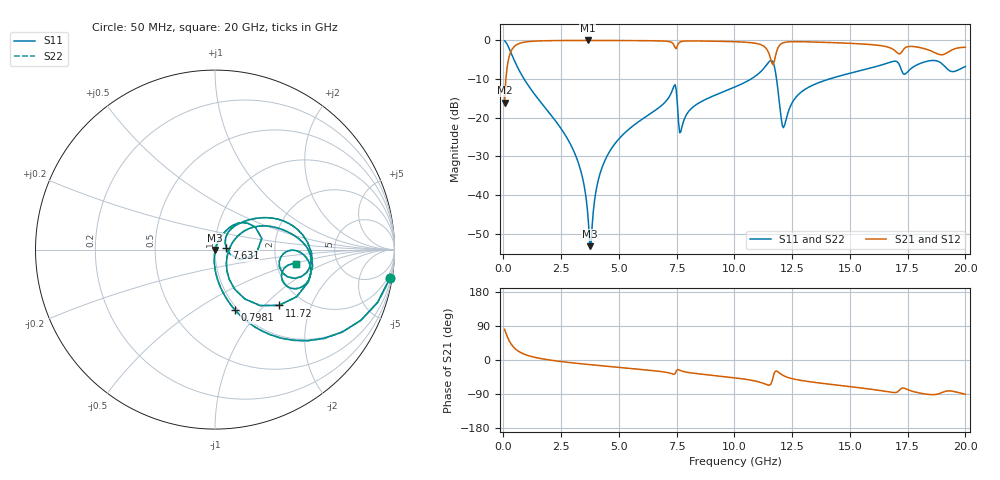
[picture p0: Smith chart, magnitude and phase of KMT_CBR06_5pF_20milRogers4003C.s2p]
! Data measured by Modelithics Inc. support@modelithics.com 813-866-6335
! KEMET CBR0603 5pF, Pad Width= 0.851mm, Pad Length= 0.64mm, Pad Gap= 0.62mm, 20mil Rogers 4003C substrate Data, January 2022
# hz S ma R 50
! 2 Port Network Data from SP1.SP block
! freq  magS11  angS11  magS21  angS21  magS12  angS12  magS22  angS22
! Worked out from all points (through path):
!   401 points, 50 MHz to 20 GHz, reference 50 ohm
!   highest |S21| = -0.02 dB at 3.641 GHz (marker M1); lowest = -16.1 dB at 50 MHz (marker M2)
!   group delay of S21, straight-line fit = 15.4 ps
!   lowest |S11| = -53.2 dB at 3.741 GHz (marker M3), VSWR 1.00, Z = 50.2 - j0.15 ohm
!   |S11| at or under -10 dB: 895.2 MHz to 10.72 GHz (9.821 GHz wide, 169 % of centre); 11.82 GHz to 14.1 GHz (2.276 GHz wide, 17.6 % of centre)
!   |S22| runs from -53.2 to -0.1 dB; largest |S21 - S12| = 0
!   S11 on the Smith chart (normalised r, x): 50 MHz: 1, -12; 798.1 MHz: 0.97, -0.74; 7.631 GHz: 1.13, +0.02; 11.72 GHz: 1.52, -1.22; 20 GHz: 2.58, -0.51
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5e7  0.9876 -9.2  0.1564 80.8  0.1564 80.8  0.9876 -9.2
2.99375e8  0.7232 -44.6  0.6899 45.3  0.6899 45.3  0.7232 -44.6
7.98125e8  0.3538 -71.8  0.9343 18.1  0.9343 18.1  0.3538 -71.8
2.693375e9  0.05858 -93.9  0.9966 -5.5  0.9966 -5.5  0.05858 -93.9
3.391625e9  0.01835 -94.5  0.9979 -10.1  0.9979 -10.1  0.01835 -94.5
3.641e9  0.006161 -84.2  0.998 -11.6  0.998 -11.6  0.006161 -84.2
3.74075e9  0.002185 -43.2  0.998 -12.2  0.998 -12.2  0.002185 -43.2
4.089875e9  0.01493 68.1  0.9978 -14.3  0.9978 -14.3  0.01493 68.1
4.53875e9  0.03419 69.6  0.9972 -16.9  0.9972 -16.9  0.03419 69.6
6.73325e9  0.1352 58.1  0.9857 -29.8  0.9857 -29.8  0.1352 58.1
7.381625e9  0.2569 29.4  0.8717 -37.8  0.8717 -37.8  0.2569 29.4
7.631e9  0.06385 7.7  0.9466 -27.0  0.9466 -27.0  0.06385 7.7
1.0025e10  0.2501 41.3  0.961 -47.1  0.961 -47.1  0.2501 41.3
1.127188e10  0.4346 19.8  0.8405 -62.0  0.8405 -62.0  0.4346 19.8
1.157112e10  0.5512 -9.7  0.5726 -64.1  0.5726 -64.1  0.5512 -9.7
1.172075e10  0.4727 -41.1  0.5283 -35.1  0.5283 -35.1  0.4727 -41.1
1.211975e10  0.07437 -14.0  0.9328 -41.1  0.9328 -41.1  0.07437 -14.0
1.336662e10  0.2615 29.4  0.9538 -58.3  0.9538 -58.3  0.2615 29.4
1.670825e10  0.518 0.2  0.8083 -84.5  0.8083 -84.5  0.518 0.2
1.735662e10  0.3641 -10.3  0.7856 -74.5  0.7856 -74.5  0.3641 -10.3
1.895262e10  0.5079 -25.2  0.6518 -86.7  0.6518 -86.7  0.5079 -25.2
2e10  0.4598 -9.8  0.815 -90.4  0.815 -90.4  0.4598 -9.8
